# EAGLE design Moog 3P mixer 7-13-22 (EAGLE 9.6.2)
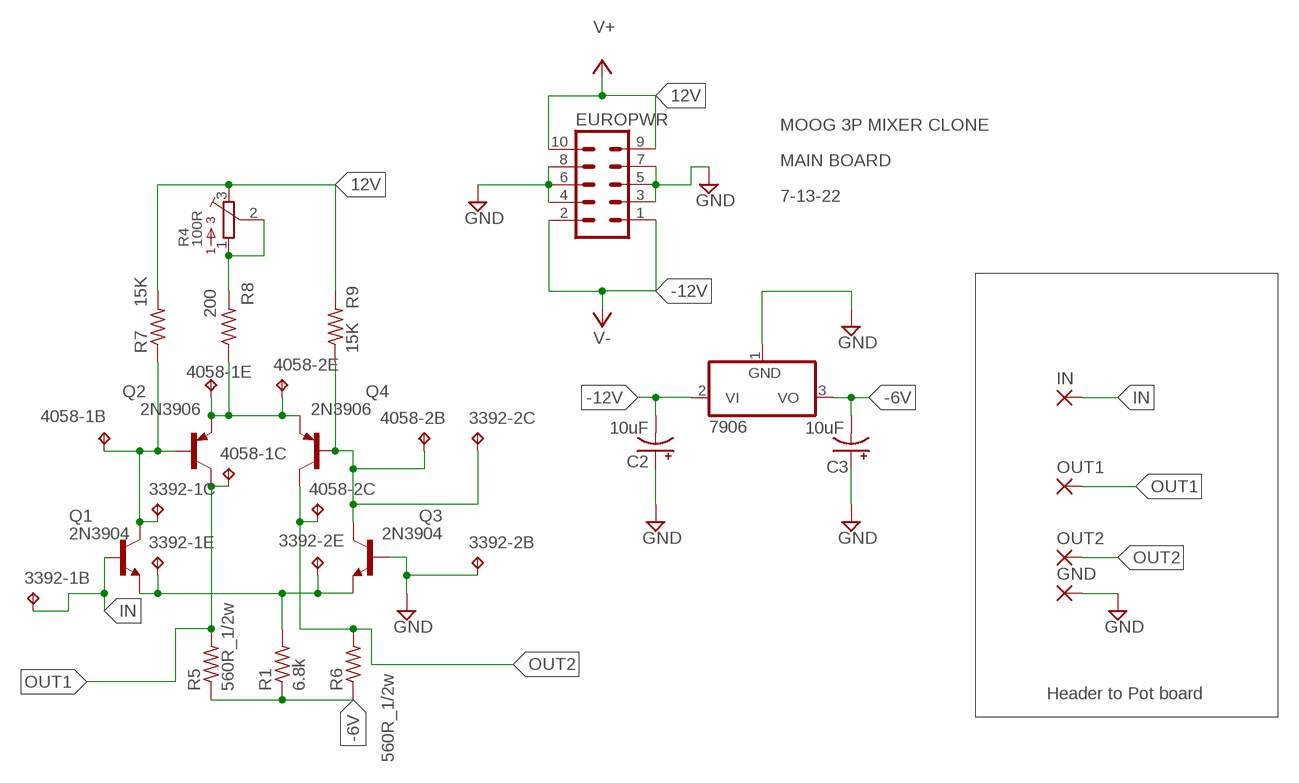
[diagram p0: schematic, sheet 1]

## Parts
3392-1B  TPPAD1-13  [P1-13]
3392-1C  TPPAD1-13  [P1-13]
3392-1E  TPPAD1-13  [P1-13]
3392-2B  TPPAD1-13  [P1-13]
3392-2C  TPPAD1-13  [P1-13]
3392-2E  TPPAD1-13  [P1-13]
4058-1B  TPPAD1-13  [P1-13]
4058-1C  TPPAD1-13  [P1-13]
4058-1E  TPPAD1-13  [P1-13]
4058-2B  TPPAD1-13  [P1-13]
4058-2C  TPPAD1-13  [P1-13]
4058-2E  TPPAD1-13  [P1-13]
7906  7906T  [TO220H]
C2  10uF  CPOL-USE5-8.5  [E5-8,5]
C3  10uF  CPOL-USE5-8.5  [E5-8,5]
EUROPWR  EURO_POWER_HEADERREGULAR  [EURO_POWER_HEADER]
GND  WIREPAD1,6/0,9  [1,6/0,9]
IN  WIREPAD1,6/0,9  [1,6/0,9]
OUT1  WIREPAD1,6/0,9  [1,6/0,9]
OUT2  WIREPAD1,6/0,9  [1,6/0,9]
Q1  2N3904  [TO92]
Q2  2N3906  [TO92]
Q3  2N3904  [TO92]
Q4  2N3906  [TO92]
R1  6.8k  R-US_0204/7  [0204/7]
R4  100R  3386-X  [3386X]
R5  560R_1/2w  R-US_0617/22  [0617/22]
R6  560R_1/2w  R-US_0617/22  [0617/22]
R7  15K  R-US_0204/7  [0204/7]
R8  200  R-US_0204/7  [0204/7]
R9  15K  R-US_0204/7  [0204/7]

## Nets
12V: EUROPWR.9 EUROPWR.10 R4.3 R7.2 R9.2 ; supply symbol labelled V+
-6V: 7906.3(VO) C3.- R1.1 R5.1 R6.1
-12V: 7906.2(VI) C2.- EUROPWR.1 EUROPWR.2 ; supply symbol labelled V-
GND: 3392-2B.TP 7906.1(GND) C2.+ C3.+ EUROPWR.3 EUROPWR.4 EUROPWR.5 EUROPWR.6 EUROPWR.7 EUROPWR.8 GND.1(P) Q3.2(B)
IN: 3392-1B.TP IN.1(P) Q1.2(B)
N$1: 3392-1E.TP 3392-2E.TP Q1.3(E) Q3.3(E) R1.2
N$2: 4058-1E.TP 4058-2E.TP Q2.3(E) Q4.3(E) R8.1
N$5: 3392-1C.TP 4058-1B.TP Q1.1(C) Q2.2(B) R7.1
N$6: 3392-2C.TP 4058-2B.TP Q3.1(C) Q4.2(B) R9.1
N$7: R4.1 R4.2 R8.2
OUT1: 4058-1C.TP OUT1.1(P) Q2.1(C) R5.2
OUT2: 4058-2C.TP OUT2.1(P) Q4.1(C) R6.2

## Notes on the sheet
- MOOG 3P MIXER CLONE
- MAIN BOARD
- 7-13-22
- Header to Pot board

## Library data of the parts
3392-1B 3392-1C 3392-1E 3392-2B 3392-2C 3392-2E 4058-1B 4058-1C 4058-1E 4058-2B 4058-2C 4058-2E = testpad:TP: Test pad
7906 = linear:79*: Negative VOLTAGE REGULATOR
C2 C3 = rcl:CPOL-US: POLARIZED CAPACITOR, American symbol; SPICEPREFIX: C
EUROPWR = MusicThingModular:EURO_POWER_HEADER: Power Header 10 pin power header for Eurorack Power Supplies Variants with fatter pads for easier soldering, and the LOCK variant which has 5mil offset pins to hold the component in place before soldering
GND IN OUT1 OUT2 = wirepad:WIREPAD: Wire PAD connect wire on PCB
Q1 Q3 = transistor-npn:2N3904: NPN Transistor
Q2 Q4 = transistor-pnp:2N3906: PNP Transistor
R1 R7-R9 = rcl:R-US_: RESISTOR, American symbol
R4 = bourns:3386-: 3386 Series 3/8" Square Trimmer
R5 R6 = rcl:R-US_: RESISTOR, American symbol; SPICEPREFIX: R

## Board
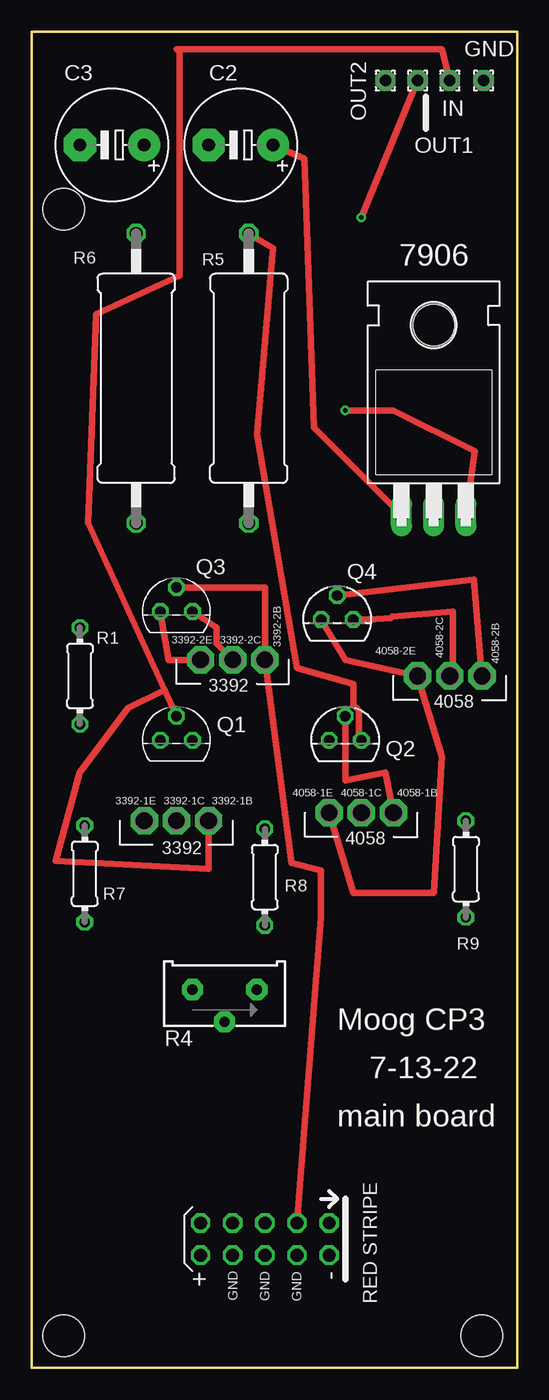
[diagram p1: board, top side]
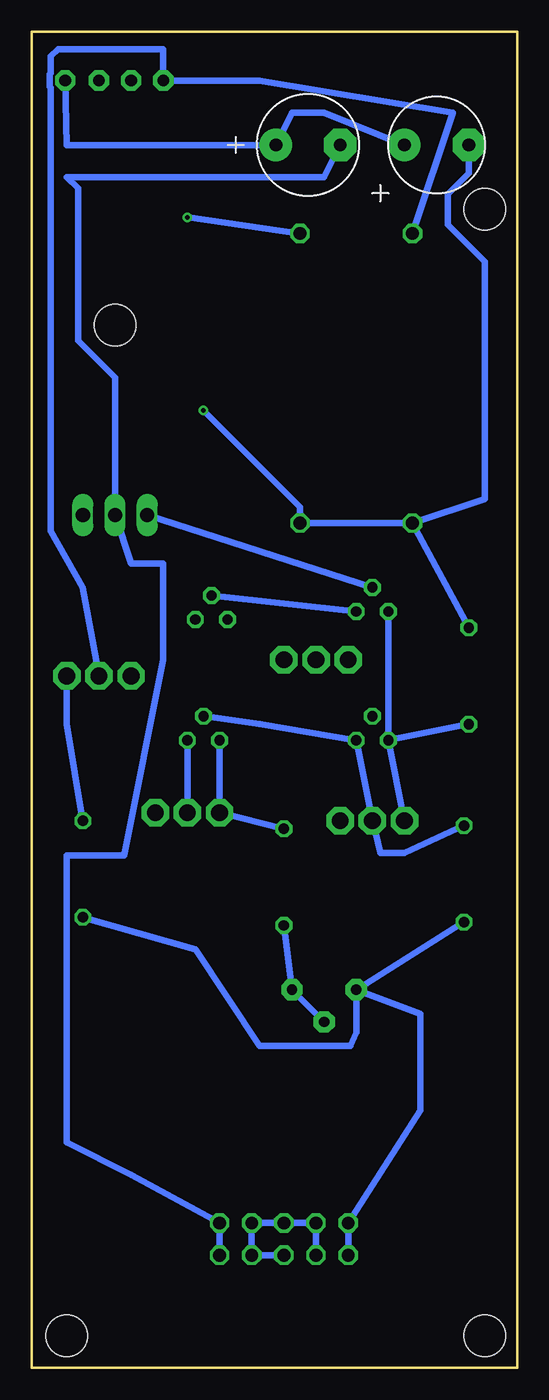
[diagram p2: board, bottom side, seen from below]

Size 38.33 x 105.46 mm. Coordinates in mm from the lower left corner, seen from the top.
Outline: 0,0 38.33,0 38.33,105.46 0,105.46 0,0
Copper layers (1*16): Top 0.035mm / dielectric 1.5mm / Bottom 0.035mm
Design rules "default": minimum track width 6mil, minimum drill 0.35mm, track to track 6mil, track to pad 6mil, pad to pad 6mil, via to via 6mil, smd to smd 6mil, copper to edge 40mil, drill to drill 6mil, minimum pad ring 10mil, minimum via ring 8mil, stop-mask expansion 4mil, vias tented up to drill 0mil, thermal gap 10mil
Holes 3.3 mm at 2.54,2.54 35.56,2.54 2.54,91.44

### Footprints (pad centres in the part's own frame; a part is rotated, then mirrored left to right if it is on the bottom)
P1-13 = drill 1.321 pad 2.159 octagon: TP 0,0
TO220H = drill 1.118 long: 1 -2.54,-10.16; 2 0,-10.16; 3 2.54,-10.16 | hole 3.302: 0,4.826
E5-8,5 = drill 1.016 pad 2.54: + -2.54,0 | drill 1.016 pad 2.54 octagon: - 2.54,0
EURO_POWER_HEADER = drill 1.016 octagon: 1 -5.08,-1.27; 2 -5.08,1.27; 3 -2.54,-1.27; 4 -2.54,1.27; 5 0,-1.27; 6 0,1.27; 7 2.54,-1.27; 8 2.54,1.27; 9 5.08,-1.27; 10 5.08,1.27
1,6/0,9 = drill 0.914 pad 1.6 octagon: 1 0,0
TO92 = drill 0.813 octagon: 1 1.27,0; 2 0,1.905; 3 -1.27,0
0204/7 = drill 0.813 octagon: 1 -3.81,0; 2 3.81,0
3386X = drill 0.813 pad 1.676 octagon: 1 2.54,0.635; 2 0,-1.905; 3 -2.54,0.635
0617/22 = drill 1.016 octagon: 1 -11.43,0; 2 11.43,0

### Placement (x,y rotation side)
3392-1B  13.97,43.18 0 top
3392-1C  11.43,43.18 0 top
3392-1E  8.89,43.18 0 top
3392-2B  18.41,55.88 0 top
3392-2C  15.88,55.88 0 top
3392-2E  13.34,55.88 0 top
4058-1B  28.57,43.81 0 top
4058-1C  26.04,43.81 0 top
4058-1E  23.5,43.81 0 top
4058-2B  35.56,54.61 0 top
4058-2C  33.02,54.61 0 top
4058-2E  30.48,54.61 0 top
7906  31.75,77.47 0 top
C2  16.51,96.52 180 top
C3  6.35,96.52 180 top
EUROPWR  18.41,10.16 180 top
GND  35.69,101.6 0 top
IN  33.02,101.6 90 top
OUT1  30.48,101.6 0 top
OUT2  27.94,101.6 0 top
Q1  11.43,49.53 0 top
Q2  24.77,49.53 0 top
Q3  11.43,59.69 0 top
Q4  24.13,59.05 0 top
R1  3.81,54.61 270 top
R4  15.24,29.21 0 top
R5  17.14,78.11 90 top
R6  8.26,78.11 90 top
R7  4.19,38.99 270 top
R8  18.41,38.73 270 top
R9  34.29,39.37 270 top

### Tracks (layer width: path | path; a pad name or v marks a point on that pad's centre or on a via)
12V
  Bottom 0.508: R4.3 R7.2 | EUROPWR.10 EUROPWR.9 7.62,20.32 7.62,27.94 R4.3 | R9.2 25.4,33.02 20.32,25.4 13.15,25.4 12.7,26.46 R4.3
-6V  (via drill 0.35)
  Top 0.508: v24.77,75.56 28.57,75.56 35.01,72.35 7906.3
  Bottom 0.508: R1.1 R6.1 | R6.1 2.54,68.58 2.54,87.31 5.46,90.23 5.46,92.65 3.81,94.3 C3.- | R6.1 R5.1 17.14,67.94 v24.77,75.56
-12V
  Bottom 0.508: EUROPWR.2 EUROPWR.1 30.48,15.24 35.56,17.78 35.56,40.44 31.03,40.44 27.94,55.88 27.94,63.5 30.48,63.5 7906.2 31.75,78.17 34.67,81.09 34.67,93.09 35.56,93.98 15.24,93.98 C2.-
GND
  Top 0.508: 7906.1 22.29,74.23 21.56,95.44 C2.+ | Q3.2 18.41,61.59 3392-2B.TP 20.5,39.86 22.86,39.27 22.86,35.56 EUROPWR.3
  Bottom 0.508: C3.+ 15.24,99.06 17.78,99.06 C2.+ 35.56,96.52 GND.1 | Q3.2 7906.1 | EUROPWR.8 EUROPWR.7 EUROPWR.5 EUROPWR.3 EUROPWR.4 EUROPWR.6
IN
  Top 0.508: Q1.2 10.49,53.49 | 10.49,53.49 4.45,66.67 5.08,83.19 11.68,86.19 11.68,103.83 11.43,104.09 32.38,104.09 IN.1 | 3392-1B.TP 13.97,39.37 1.91,40.01 3.81,46.99 7.62,52.07 10.49,53.49
N$1
  Top 0.508: 3392-2E.TP 10.79,55.88 Q3.3
  Bottom 0.508: Q1.3 9.92,49.58 R1.2 | Q1.3 Q3.3 | 3392-1E.TP Q1.3
N$2
  Top 0.508: Q4.3 24.77,55.88 4058-2E.TP 32.38,48.26 31.75,37.47 25.4,37.47 4058-1E.TP
  Bottom 0.508: R8.1 4058-1E.TP Q2.3
N$5
  Top 0.508: 4058-1B.TP 27.94,46.99 24.77,46.35 Q2.2
  Bottom 0.508: Q2.2 20.32,50.8 Q1.1 11.55,43.79 | 3392-1C.TP 11.55,43.79 | R7.1 8.89,40.64 10.79,40.64 11.55,43.79
N$6
  Top 0.508: 4058-2B.TP 34.92,62.23 Q4.2 | 3392-2C.TP 14.61,57.15 14.61,58.42 Q3.1
  Bottom 0.508: R9.1 35.56,50.8 4058-2B.TP | Q3.1 Q4.2
N$7
  Bottom 0.508: R8.2 R4.1 R4.2
OUT1  (via drill 0.35)
  Top 0.508: v26.04,90.81 OUT1.1 | R5.2 19.05,88.39 17.78,73.66 20.95,55.24 25.4,53.98 25.4,52.31 25.83,51.88 25.83,49.73 Q2.1
  Bottom 0.508: R5.2 v26.04,90.81 | 4058-1C.TP Q2.1
OUT2
  Top 0.508: 4058-2C.TP 33.27,54.86 33.27,59.71 28.48,59.31 28.37,59.2 26.67,59.05 Q4.1
  Bottom 0.508: R6.2 5.08,99.06 20.32,101.6 OUT2.1 27.94,104.09 36.25,104.09 36.83,103.5 36.83,102.16 36.89,102.1 36.89,101.1 36.83,101.04 36.83,66.04 34.29,61.59 4058-2C.TP

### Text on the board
tNames: 3392 | 4058 | 3392 | 4058 | Moog CP3 | 7-13-22 | main board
